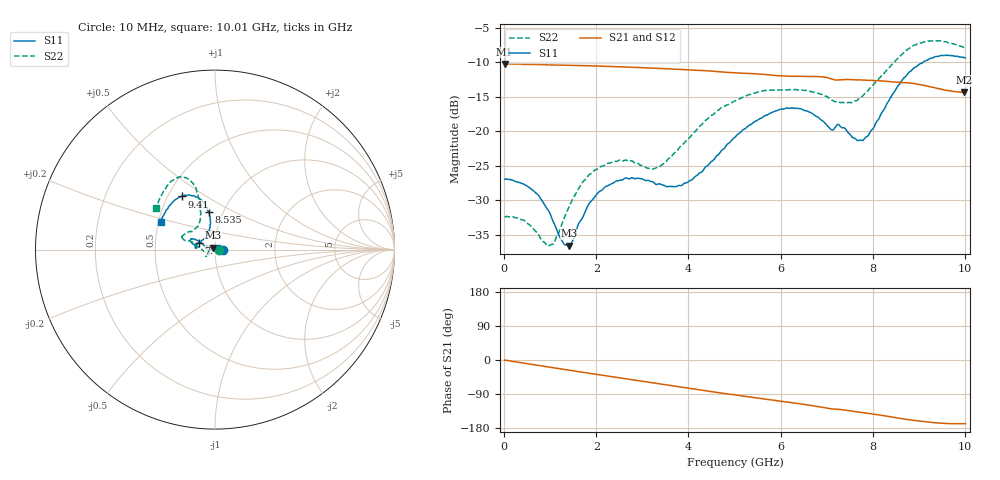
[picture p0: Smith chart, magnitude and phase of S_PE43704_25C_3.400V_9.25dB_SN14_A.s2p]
! Device ID: PE43704
! Dir: z:\PE43704\PE43704_Char_1_20130516\PE43704\AMB\3p400V\9p25dB
! Serial: 14
! Insertion: A
! Impedance: 50 ohm
! Temp: Amb
! VDD: 3.400V
! Attenuation Step: 9.25dB
! IDD: 1.140853e-01mA
#  Hz  S  RI  R  50
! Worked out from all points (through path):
!   401 points, 10 MHz to 10.01 GHz, reference 50 ohm
!   highest |S21| = -10.25 dB at 10 MHz (marker M1); lowest = -14.4 dB at 9.985 GHz (marker M2)
!   group delay of S21, straight-line fit = 48.5 ps
!   lowest |S11| = -36.6 dB at 1.41 GHz (marker M3), VSWR 1.03, Z = 48.9 + j0.981 ohm
!   |S11| at or under -10 dB: start of sweep to 9.096 GHz
!   |S22| runs from -36.7 to -6.8 dB; largest |S21 - S12| = 0.0024
!   S11 on the Smith chart (normalised r, x): 10 MHz: 1.09, +0.00; 7.46 GHz: 0.83, +0.07; 8.535 GHz: 0.86, +0.37; 9.41 GHz: 0.59, +0.40; 10.01 GHz: 0.51, +0.18
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1e7  0.0448 0.000279  0.3073 -0.00116  0.3073 -0.00116  0.0239 0.000276
5.85e8  0.0322 0.0205  0.2987 -0.0598  0.2986 -0.0597  0.0127 0.0161
9.85e8  0.0127 0.0224  0.2867 -0.0978  0.2867 -0.0977  -0.00577 0.0137
1.26e9  -0.00267 0.0157  0.2753 -0.1231  0.2753 -0.123  -0.0211 0.00466
1.41e9  -0.0108 0.01  0.2681 -0.1359  0.2682 -0.1358  -0.0284 -0.00227
1.685e9  -0.0231 -0.000887  0.2535 -0.1586  0.2535 -0.1584  -0.0388 -0.0156
2.01e9  -0.0324 -0.013  0.2335 -0.183  0.2336 -0.1828  -0.0442 -0.0289
2.41e9  -0.0359 -0.0238  0.2058 -0.2094  0.206 -0.2092  -0.0481 -0.0366
3.36e9  -0.0346 -0.0231  0.1301 -0.2537  0.1303 -0.2535  -0.052 -0.0174
4.035e9  -0.0439 0.000131  0.0715 -0.2683  0.0719 -0.2684  -0.0897 0.0126
5.01e9  -0.0809 0.0403  -0.01 -0.2647  -0.00989 -0.2649  -0.1585 0.0492
5.96e9  -0.1291 0.0605  -0.0783 -0.2402  -0.0774 -0.2404  -0.1876 0.0654
6.685e9  -0.1295 0.0369  -0.1264 -0.2147  -0.1264 -0.2144  -0.1751 0.0817
7.085e9  -0.1018 0.0172  -0.1505 -0.1876  -0.151 -0.1881  -0.1368 0.101
7.46e9  -0.0898 0.0391  -0.163 -0.1721  -0.1624 -0.1722  -0.1035 0.1236
7.835e9  -0.0492 0.0748  -0.1791 -0.1512  -0.1789 -0.1517  -0.0826 0.1699
8.36e9  -0.0264 0.1667  -0.1968 -0.1164  -0.1961 -0.1175  -0.0869 0.276
8.535e9  -0.0357 0.2076  -0.2017 -0.1033  -0.2002 -0.1042  -0.1011 0.3204
8.91e9  -0.0804 0.2791  -0.2073 -0.0773  -0.2065 -0.0761  -0.1507 0.3938
9.41e9  -0.1825 0.2962  -0.1983 -0.0489  -0.1981 -0.0481  -0.2307 0.388
9.985e9  -0.2981 0.1642  -0.1872 -0.0391  -0.188 -0.0388  -0.3227 0.2385
1.001e10  -0.303 0.154  -0.1879 -0.0397  -0.1889 -0.0398  -0.3261 0.2304
